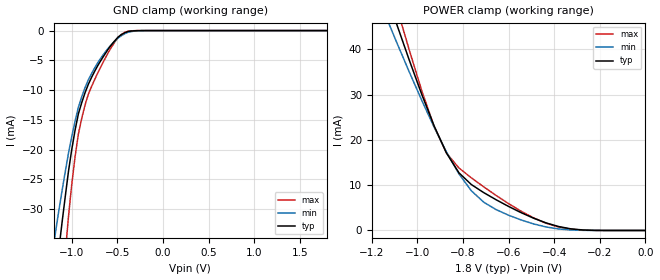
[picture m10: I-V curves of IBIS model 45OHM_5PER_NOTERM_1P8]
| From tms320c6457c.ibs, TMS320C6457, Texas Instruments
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|   Model Cell 45OHM_5PER_NOTERM_1P8
|45OHM_5PER_NOTERM_1P8
[Model]   45OHM_5PER_NOTERM_1P8
Model_type   Input
Polarity   Non-Inverting
Vinl =  0.8
Vinh =  1
C_comp   1.89p   1.72p   2.18p
[Model Spec]
Vinl   0.8   0.755   0.845
Vinh   1   0.955   1.045
D_overshoot_high 2.34 NA NA
D_overshoot_low -0.54 NA NA
D_overshoot_time 0.56n NA NA
S_overshoot_high 2.2 NA NA
S_overshoot_low -0.4 NA NA
[Receiver Thresholds]
Vth = 0.9V
Vth_min = 0.855V
Vth_max = 0.945V
Vinl_dc = -125mV
Vinh_dc = +125mV
Vinl_ac = -250mV
Vinh_ac = +250mV
Tslew_ac = 5.000ns
Threshold_sensitivity = 0.50
Reference_supply Pullup_ref
[Temperature Range]   25   125   -40
[Voltage Range]   1.8   1.71   1.89
[Pullup reference]   1.8   1.71   1.89
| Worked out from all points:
|   GND clamp passes 1 mA (typ) near -0.48 V on its own axis
|   POWER clamp passes 1 mA (typ) near -0.39 V on its own axis
[POWER_clamp]
|   voltage   I(typ)   I(min)   I(max)
-1.8V     156mA      133.5mA    181.7mA
-1.127V   50.87mA    45.88mA    55.74mA
-1.109V   48.19mA    43.68mA    52.51mA
-1.073V   42.88mA    39.33mA    46.15mA
-1.055V   40.27mA    37.18mA    43.01mA
-927.3mV  23.11mA    22.83mA    22.99mA
-872.7mV  17.08mA    17.31mA    17.08mA
-818.2mV  12.73mA    12.5mA     13.8mA
-763.6mV  10.13mA    8.758mA    11.61mA
-600mV    5.297mA    3.36mA     5.91mA
-381.8mV  881.1uA    335uA      768.7uA
0V        130.3nA    168.6nA    304.6nA
[GND_clamp]
|   voltage   I(typ)   I(min)   I(max)
-1.8V     -137.1mA   -107.1mA   -189.7mA
-1.182V   -42.18mA   -34.28mA   -58.62mA
-1.109V   -32.61mA   -27.18mA   -44.51mA
-1.073V   -28.08mA   -23.86mA   -37.8mA
-1.036V   -23.72mA   -20.65mA   -31.33mA
-963.6mV  -16.74mA   -15.21mA   -21.21mA
-927.3mV  -13.99mA   -12.88mA   -17.37mA
-854.5mV  -10.47mA   -9.599mA   -12.54mA
-781.8mV  -7.837mA   -7.199mA   -9.372mA
-600mV    -3.116mA   -2.961mA   -3.703mA
-418.2mV  -354.7uA   -522.5uA   -297.2uA
1.8V      130.3nA    376.5nA    216.8nA
